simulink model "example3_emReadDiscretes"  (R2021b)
settings: Solver=FixedStepAuto  StartTime=0  StopTime=inf  FixedStep=0.5  RelTol=1e-3  EnableMultiTasking=on
undefined symbols (not defined in the file or in its folder): based, classic, dsPic33, MCC, Microchip, PIC24
libraries: emMBSlaveLib x2, embeddedCreatorLib x1

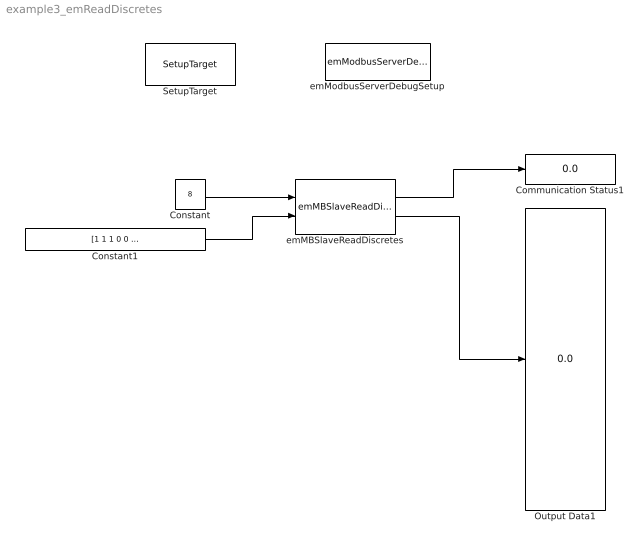
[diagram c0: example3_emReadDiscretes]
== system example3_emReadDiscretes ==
  Communication Status1 : Display
  Constant : Constant  Value=8  OutDataTypeStr=uint16
  Constant1 : Constant  Value=[1 1 1 0 0 0 1 1 1 0 0 0 1 1 1 1 1]  OutDataTypeStr=boolean
  Output Data1 : Display
  SetupTarget : embeddedCreatorLib/SetupTarget  Tag=SetupTarget  Priority=0  c_platform=Microchip PIC24/dsPic33 based on MCC classic  c_debug=on
  emMBSlaveReadDiscretes : emMBSlaveLib/emMBSlaveReadDiscretes  c_ServerID=1  c_minAdr=8  c_RegQTY=18  c_sampleTime=-1
  emModbusServerDebugSetup : emMBSlaveLib/emModbusServerDebugSetup  Tag=emModbusSlaveSetup  c_objID=0  c_uartNo=2  c_baudrate=19200  c_serverID=1  c_baudrate4PC=19200  c_forceLongerSpace=on  c_holdingRegsQTY=0  c_minHoldingAddr=789  c_inputRegsQTY=0  c_minInputRegAddr=1  c_coilRegsQTY=0  c_minCoilAddr=30  c_discreteRegsQTY=18  c_minDiscreteAddr=8  c_enableDebug=on  c_breakpointMaxQTY=100  c_probeMaxWordQTY=200  c_emWaitQTY=0  g_COMPortNo=COM5  c_Name_method=By physical port name and bit number  c_PortName=B  c_BitNo=11  c_TxEnable485="\"LATBbits.LATB11\""  c_TxEnable485Polarity=on
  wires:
  Constant/1 -> emMBSlaveReadDiscretes/1
  emMBSlaveReadDiscretes/1 -> Communication Status1/1
  emMBSlaveReadDiscretes/2 -> Output Data1/1
  Constant1/1 -> emMBSlaveReadDiscretes/2
